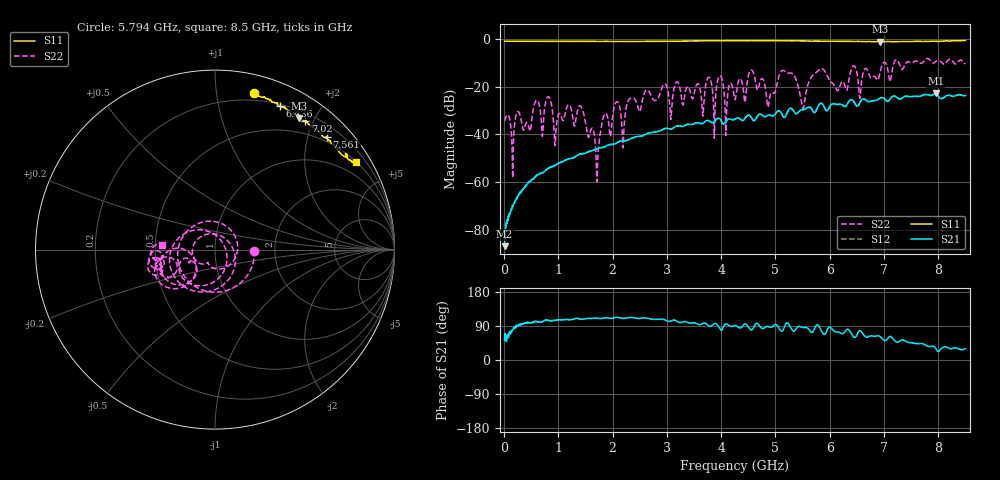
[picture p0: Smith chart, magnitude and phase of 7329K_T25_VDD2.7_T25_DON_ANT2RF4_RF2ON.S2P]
!Agilent Technologies,E5071C,MY46417908,A.11.23
!Date: Mon Aug 31 18:03:11 2020
!Data & Calibration Information:
!Freq	S11:SOLT2(ON)	S21:SOLT2(ON)	S12:SOLT2(ON)	S22:SOLT2(ON)
!PortZ  Port1:50+j0  Port2:50+j0
!Above PortZ is port z conversion or system Z0 setting when saving the data.
!When reading, reference impedance value at option line is always used.
# Hz S dB R 50
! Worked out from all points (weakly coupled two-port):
!   1601 points, 10 MHz to 8.5 GHz, reference 50 ohm
!   highest |S21| = -22.79 dB at 7.953 GHz (marker M1); lowest = -86.9 dB at 10 MHz (marker M2)
!   lowest |S11| = -1.2 dB at 6.924 GHz (marker M3), VSWR 14.45, Z = 14.8 + j89.7 ohm
!   |S11| at or under -10 dB: nowhere
!   |S22| runs from -59.9 to -8.2 dB; largest |S21 - S12| = 0.00081
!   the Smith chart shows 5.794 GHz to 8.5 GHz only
!   S11 on the Smith chart (normalised r, x): 5.794 GHz: 0.14, +1.27; 6.436 GHz: 0.22, +1.53; 7.02 GHz: 0.31, +1.88; 7.561 GHz: 0.40, +2.34; 8.5 GHz: 0.51, +3.44
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1e7  -0.98 179.7  -86.95 52.1  -84.96 63.9  -34.40 5.1
4.663375e8  -1.05 169.1  -60.11 98.0  -59.96 97.2  -38.09 29.7
1.426769e9  -1.06 150.8  -48.14 107.7  -48.26 107.3  -28.66 -79.2
1.718612e9  -1.08 145.0  -45.95 110.5  -45.99 110.2  -55.18 -17.5
2.068825e9  -1.10 137.9  -43.70 112.6  -43.75 112.8  -26.43 86.1
2.190869e9  -1.10 135.2  -42.81 109.7  -42.82 109.7  -45.75 51.5
2.323525e9  -1.11 132.3  -42.00 112.3  -42.00 112.3  -24.95 59.2
2.843538e9  -1.06 119.4  -38.78 107.3  -38.79 107.3  -24.68 22.8
4.255e9  -0.76 95.3  -33.63 91.0  -33.64 91.0  -25.50 -118.4
4.557456e9  -0.73 91.8  -33.12 79.3  -33.11 79.3  -13.07 -143.8
4.875831e9  -0.76 87.7  -31.98 87.5  -31.98 87.5  -27.42 -151.5
5.151756e9  -0.81 84.1  -32.90 82.1  -32.87 82.0  -13.30 150.8
5.507275e9  -0.88 79.7  -29.75 85.5  -29.72 85.6  -29.24 0.2
5.671769e9  -0.96 76.9  -29.58 72.8  -29.55 72.8  -15.74 -163.1
5.793812e9  -0.93 75.9  -27.98 90.7  -27.97 90.8  -13.19 -1.4
6.435869e9  -1.15 65.6  -26.05 61.6  -26.07 61.6  -11.32 -137.0
6.924044e9  -1.20 57.3  -24.88 62.2  -24.90 62.0  -14.40 -126.3
7.019556e9  -1.16 55.0  -25.38 51.2  -25.41 51.0  -9.89 -161.4
7.088538e9  -1.14 54.7  -25.95 60.1  -26.00 60.0  -15.39 179.8
7.560794e9  -1.06 45.3  -24.07 44.3  -24.08 44.4  -9.52 -159.1
7.953456e9  -1.06 39.4  -22.79 31.0  -22.81 31.2  -9.48 -164.2
8.5e9  -0.68 31.8  -23.71 29.9  -23.74 29.6  -10.57 175.5
